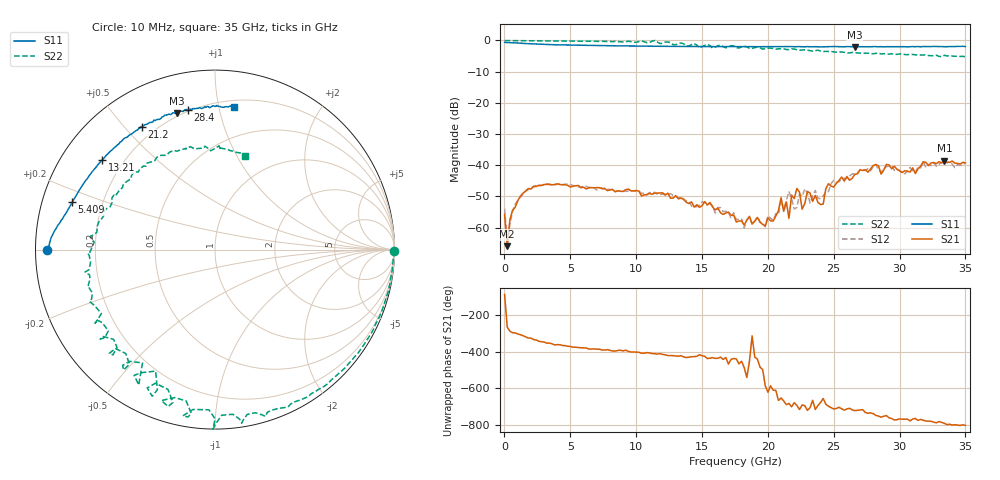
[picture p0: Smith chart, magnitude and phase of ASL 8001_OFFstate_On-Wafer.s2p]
!ASL 8001 Wideband SPST Switch
!OFF State On-Wafer S-parameter data from 10MHz-35 GHz
!Agilent Technologies,E8363B,MY43030569,A.06.01.05
!Agilent E8363B: A.06.01.05
!Date: Thursday, August 10, 2006 16:53:44
!Correction: S11(Full 2 Port(1,2)) S21(Full 2 Port(1,2)) S12(Full 2 Port(1,2)) S22(Full 2 Port(1,2))
!S2P File: Measurements: S11, S21, S12, S22:
# Hz S  dB  R 50
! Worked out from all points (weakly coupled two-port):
!   176 points, 10 MHz to 35 GHz, reference 50 ohm
!   highest |S21| = -38.57 dB at 33.4 GHz (marker M1); lowest = -66.0 dB at 209.9 MHz (marker M2)
!   lowest |S11| = -2.1 dB at 26.6 GHz (marker M3), VSWR 8.46, Z = 9.26 + j37.2 ohm
!   |S11| at or under -10 dB: nowhere
!   |S22| runs from -5.2 to 0.0 dB; largest |S21 - S12| = 0.0025
!   S11 on the Smith chart (normalised r, x): 10 MHz: 0.03, -0.00; 5.409 GHz: 0.09, +0.16; 13.21 GHz: 0.12, +0.35; 21.2 GHz: 0.15, +0.56; 28.4 GHz: 0.19, +0.81; 35 GHz: 0.25, +1.11
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1e7  -0.59 -180.0  -55.84 -88.7  -53.89 -74.6  -0.02 -0.4
2.0995e8  -0.68 178.9  -65.95 93.5  -64.85 76.6  -0.04 -1.7
6.0985e8  -0.74 176.7  -54.48 63.3  -54.80 68.1  -0.05 -4.9
1.80955e9  -1.02 171.6  -47.46 34.1  -47.82 37.6  -0.06 -14.1
5.40865e9  -1.54 161.7  -46.58 -15.2  -46.53 -16.4  -0.18 -42.1
6.0085e9  -1.58 160.1  -47.05 -19.5  -46.74 -20.4  -0.22 -46.7
1.180705e10  -1.87 145.0  -48.87 -50.5  -49.39 -48.8  -0.98 -92.2
1.32067e10  -1.91 141.4  -50.76 -64.3  -50.55 -62.4  -0.99 -109.6
1.76056e10  -1.96 130.0  -58.20 -79.7  -57.44 -94.5  -2.25 -135.0
1.980505e10  -1.99 124.0  -59.45 133.7  -59.76 121.7  -2.64 -154.7
2.100475e10  -1.94 121.0  -50.43 67.6  -51.34 56.4  -2.62 -164.0
2.12047e10  -1.99 120.7  -54.80 51.5  -54.11 35.5  -2.67 -164.1
2.16046e10  -1.96 119.3  -57.05 37.9  -48.45 27.3  -2.94 -168.6
2.220445e10  -1.98 117.7  -47.44 27.5  -53.53 20.1  -2.97 -171.0
2.260435e10  -2.02 116.5  -54.08 29.5  -50.01 8.9  -3.08 -177.3
2.300425e10  -1.96 115.2  -48.41 0.2  -49.01 17.7  -3.10 -178.3
2.340415e10  -2.01 114.3  -51.60 54.8  -49.79 16.0  -3.42 176.5
2.660335e10  -2.06 105.5  -42.94 -1.3  -42.79 -1.3  -3.89 151.6
2.84029e10  -2.02 100.9  -40.19 -31.2  -41.51 -36.4  -4.07 136.2
2.92027e10  -2.01 98.3  -39.92 -40.1  -40.27 -41.5  -4.39 129.7
3.340165e10  -1.99 87.5  -38.57 -70.1  -38.39 -70.0  -4.76 87.7
3.500125e10  -1.95 82.3  -39.25 -81.7  -39.32 -83.1  -5.22 72.0
